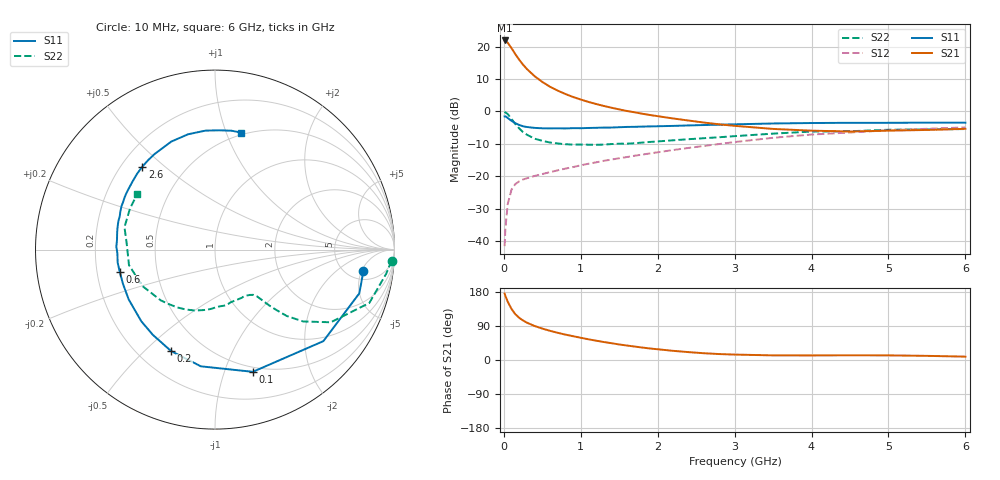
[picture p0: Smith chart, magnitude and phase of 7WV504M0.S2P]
! Infineon Technologies  Discrete & RF Semiconductors
! BFS17W
! Si NPN RF Bipolar Junction Transistor in SOT323
! VCE = 0.5 V  IC = 4 mA
! Common Emitter S-Parameters:  August  1999
# GHz  S  MA  R  50
!  f  S11  S21  S12  S22
! GHz  MAG  ANG  MAG  ANG  MAG  ANG  MAG  ANG
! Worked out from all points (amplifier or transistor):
!   36 points, 10 MHz to 6 GHz, reference 50 ohm
!   highest |S21| = 21.9 dB at 10 MHz (marker M1)
!   |S21| within 3 dB of that: start of sweep to 116.5 MHz
!   unconditionally stable (mu >= 1): 506.9 MHz to end of sweep
!   at 250 MHz: K = 0.58, MSG = 17.7 dB, |S12| = -21.0 dB
!   at 1.4 GHz: K = 1.44, MAG = 4.1 dB, |S12| = -14.9 dB
!   at 6 GHz: K = 1.15, MAG = -2.5 dB, |S12| = -4.9 dB
!   S11 on the Smith chart (normalised r, x): 10 MHz: 6.78, -5.42; 100 MHz: 0.45, -1.25; 200 MHz: 0.33, -0.61; 600 MHz: 0.30, -0.11; 2.6 GHz: 0.28, +0.42; 6 GHz: 0.48, +1.13
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0.01  0.8356 -8.3  12.41 175.2  0.0083 84.5  0.9864 -3.6
0.02  0.8401 -16.9  12.37 169.2  0.0154 82.6  0.9627 -8.1
0.05  0.7903 -40.2  11.44 154.1  0.0369 69.5  0.9097 -19.1
0.1  0.7128 -72.8  9.427 134.6  0.0621 54.8  0.7619 -32.1
0.15  0.6551 -96.9  7.607 120.7  0.0756 45.8  0.6335 -39.2
0.2  0.616 -113.4  6.251 111.3  0.0831 41.5  0.5437 -42.8
0.25  0.5878 -126.1  5.236 104.2  0.0888 38.6  0.4776 -44.6
0.3  0.5728 -135.8  4.493 98.5  0.0928 38.1  0.4356 -45.8
0.4  0.5553 -150.0  3.483 89.7  0.1006 37.7  0.3783 -47.2
0.5  0.5472 -159.5  2.841 82.9  0.1078 38.7  0.3503 -48.1
0.6  0.545 -166.7  2.396 77.0  0.1151 40.2  0.3302 -49.8
0.7  0.5472 -172.5  2.087 71.8  0.1228 41.8  0.319 -52.3
0.8  0.5442 -177.7  1.851 67.0  0.1306 42.8  0.3111 -55.3
1.1  0.5535 170.0  1.397 54.6  0.1553 45.7  0.3055 -65.3
1.3  0.5615 163.4  1.21 47.4  0.1723 46.8  0.3064 -73.3
1.6  0.5744 155.1  1.012 38.2  0.197 47.8  0.317 -85.0
2.2  0.5958 140.4  0.776 24.2  0.2528 48.4  0.3573 -108.2
2.6  0.6143 131.3  0.671 17.9  0.2922 47.3  0.3846 -123.1
3.5  0.6493 112.0  0.535 12.2  0.3905 41.4  0.4527 -153.4
4.5  0.6651 94.5  0.488 12.4  0.4713 30.8  0.4926 176.4
5.5  0.6688 82.1  0.516 10.9  0.5378 21.2  0.5261 154.2
6  0.6677 77.4  0.537 8.9  0.5656 16.5  0.5323 144.5
